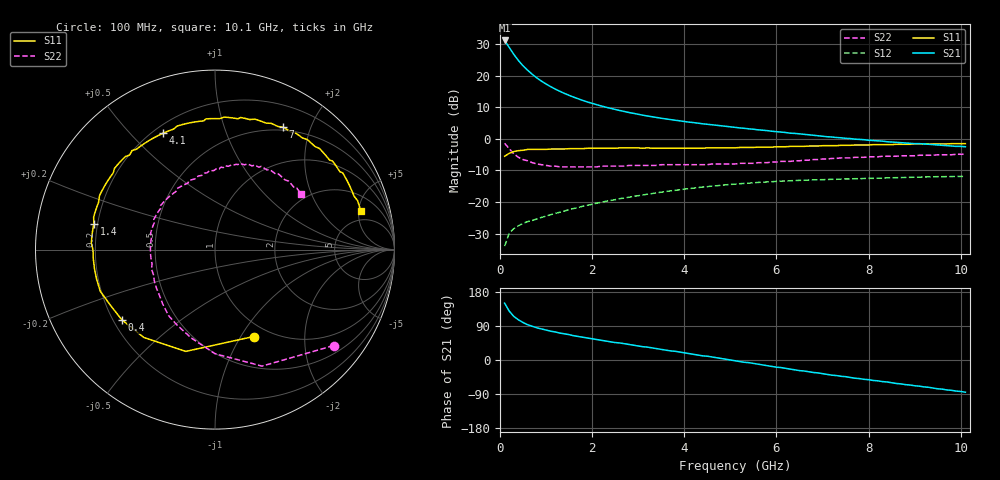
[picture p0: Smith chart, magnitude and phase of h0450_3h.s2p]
!HBFP-0450
!S and NOISE PARAMETERS at Vce=3V  Ic=50mA.  LAST UPDATED  09-04-98
# GHZ S MA R  50
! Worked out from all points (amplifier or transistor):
!   101 points, 100 MHz to 10.1 GHz, reference 50 ohm
!   highest |S21| = 31.2 dB at 100 MHz (marker M1)
!   |S21| within 3 dB of that: start of sweep to 235.8 MHz
!   unconditionally stable (mu >= 1): 2.246 GHz to end of sweep
!   at 1.7 GHz: K = 0.94, MSG = 17.2 dB, |S12| = -21.7 dB
!   at 5.1 GHz: K = 1.10, MAG = 7.1 dB, |S12| = -14.3 dB
!   at 10.1 GHz: K = 1.07, MAG = 3.1 dB, |S12| = -11.9 dB
!   lowest NFmin = 1.70 dB at 1.8 GHz
!   S11 on the Smith chart (normalised r, x): 100 MHz: 0.85, -1.14; 400 MHz: 0.23, -0.32; 1.4 GHz: 0.19, +0.10; 4.1 GHz: 0.24, +0.62; 7 GHz: 0.46, +1.60; 10.1 GHz: 3.55, +5.25
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0.1  0.53 -66.0  36.12 150.0  0.02 64.0  0.85 -39.0
0.2  0.59 -106.0  28.01 129.0  0.032 51.0  0.7 -68.0
0.3  0.63 -129.0  21.72 115.0  0.038 43.0  0.58 -90.0
0.4  0.65 -143.0  17.37 106.0  0.042 40.0  0.51 -105.0
0.5  0.66 -152.0  14.33 99.0  0.046 39.0  0.47 -117.0
0.6  0.68 -160.0  12.21 93.0  0.049 38.0  0.45 -125.0
0.7  0.68 -166.0  10.52 89.0  0.051 38.0  0.42 -134.0
0.8  0.68 -171.0  9.22 85.0  0.054 38.0  0.4 -141.0
0.9  0.68 -176.0  8.2 82.0  0.057 39.0  0.39 -147.0
1  0.68 -180.0  7.38 79.0  0.06 39.0  0.38 -153.0
1.2  0.69 174.0  6.13 74.0  0.066 40.0  0.37 -163.0
1.4  0.69 168.0  5.24 69.0  0.072 40.0  0.36 -171.0
1.8  0.7 158.0  4.05 60.0  0.086 39.0  0.36 176.0
2.1  0.71 151.0  3.47 54.0  0.096 37.0  0.36 169.0
2.5  0.71 143.0  2.92 46.0  0.109 34.0  0.37 160.0
3.5  0.71 125.0  2.12 28.0  0.143 24.0  0.39 141.0
4.1  0.71 114.0  1.84 17.0  0.163 17.0  0.39 131.0
5.1  0.72 95.0  1.52 -2.0  0.192 3.0  0.4 112.0
6.8  0.77 65.0  1.14 -33.0  0.224 -22.0  0.47 83.0
7  0.78 61.0  1.1 -36.0  0.226 -25.0  0.48 79.0
8.5  0.81 38.0  0.89 -60.0  0.242 -45.0  0.53 58.0
10.1  0.84 15.0  0.75 -85.0  0.254 -67.0  0.57 33.0
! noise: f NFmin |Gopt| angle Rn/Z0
1.8  1.7  0.61  -151  0.09
2  1.76  0.6  -149  0.11
2.5  1.9  0.61  -139  0.17
3.5  2.18  0.64  -122  0.34
4  2.33  0.66  -112  0.5
5  2.61  0.69  -93  0.88
5.5  2.76  0.72  -83  1.21
7  3.18  0.76  -57  2.4
8  3.51  0.79  -41  3.48
10  4.03  0.82  -12  5.43
